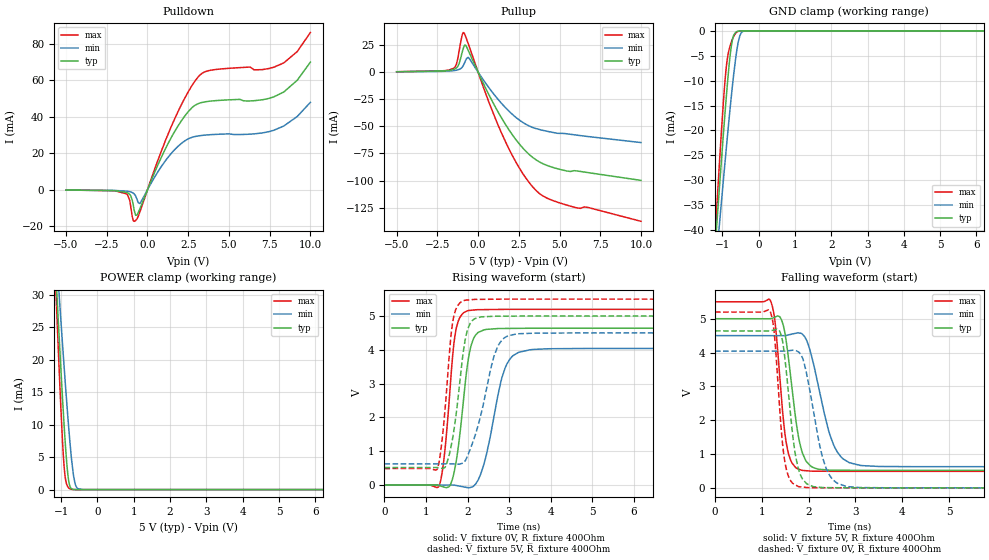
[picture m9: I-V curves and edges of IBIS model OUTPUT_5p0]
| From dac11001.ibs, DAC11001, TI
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|   OUTPUT_5p0 Model
[Model]   OUTPUT_5p0
Model_type   3-state
Polarity   Non-Inverting
Vmeas = 2.5
Vref = 0
Cref = 2pF
Rref = 100000
|   typ   min   max
C_comp   1.405pF   1.354pF   1.437pF
[Voltage Range]   5   4.5   5.5
[Temperature Range]   25   125   -40
[Pullup Reference]   5   4.5   5.5
[Pulldown Reference]   0   0   0
[Power Clamp Reference]   5   4.5   5.5
[GND Clamp Reference]   0   0   0
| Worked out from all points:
|   slope of the pulldown table from 0 to 0.75 V, typ, clamps not added: 47.3 ohm
|   slope of the pullup table from 0 to 0.75 V, typ, clamps not added: 32.1 ohm
|   GND clamp passes 1 mA (typ) near -0.69 V on its own axis
|   POWER clamp passes 1 mA (typ) near -0.78 V on its own axis
|   falling waveform, V_fixture 5V, R_fixture 400Ohm: 20-80 % time 253ps typ, 405ps min, 193ps max; typ from 5 V to 0.517 V
|   rising waveform, V_fixture 0V, R_fixture 400Ohm: 20-80 % time 262ps typ, 407ps min, 214ps max; typ from 0 V to 4.64 V
|   rising waveform, V_fixture 5V, R_fixture 400Ohm: 20-80 % time 272ps typ, 455ps min, 207ps max; typ from 0.517 V to 5 V
|   falling waveform, V_fixture 0V, R_fixture 400Ohm: 20-80 % time 222ps typ, 343ps min, 173ps max; typ from 4.64 V to 0 V
[Pulldown]
|   Voltage   I(typ)   I(min)   I(max)
-5V       -142.8uA   -116.5uA   -136.1uA
-1.25V    -1.527mA   -787.6uA   -2.341mA
-1.1V     -2.433mA   -1.025mA   -5.468mA
-875mV    -8.302mA   -1.831mA   -16.84mA
-725mV    -14.02mA   -3.432mA   -16.85mA
-455mV    -10.11mA   -7.363mA   -11.8mA
1.525V    29.73mA    20.64mA    36.03mA
2.41V     41.87mA    27.51mA    52.3mA
3.16V     47.45mA    29.62mA    62.48mA
7.75V     50.98mA    32.66mA    67.25mA
9.175V    59.95mA    40.1mA     75.72mA
10V       70.06mA    47.98mA    86.29mA
[GND Clamp]
|   Voltage   I(typ)   I(min)   I(max)
-5V       -455.7mA   -381.5mA   -546mA
-1.235V   -47.57mA   -51.99mA   -45.92mA
-1.13V    -36.77mA   -43.2mA    -32.86mA
-1.07V    -30.7mA    -38.23mA   -25.64mA
-950mV    -18.95mA   -28.46mA   -12.42mA
-875mV    -12.09mA   -22.52mA   -6.432mA
-785mV    -5.068mA   -15.68mA   -3.054mA
-725mV    -1.977mA   -11.41mA   -1.785mA
-590mV    -122.8uA   -3.502mA   -213.3uA
-485mV    -9.764uA   -489.6uA   -15.16uA
-275mV    0A         -1.303uA   0A
10V       0A         0A         0A
[Pullup]
|   Voltage   I(typ)   I(min)   I(max)
-5V       287.7uA    224.1uA    311.3uA
-1.49V    2.452mA    1.323mA    3.599mA
-1.325V   3.811mA    1.724mA    7.343mA
-1.16V    7.875mA    2.459mA    19.67mA
-965mV    18.82mA    4.665mA    34.63mA
-860mV    23.79mA    7.416mA    36.14mA
-575mV    19.02mA    13.11mA    24.9mA
1.48V     -43.28mA   -29.51mA   -57.5mA
2.365V    -63.08mA   -42.28mA   -84.07mA
3.37V     -78.83mA   -51.13mA   -106.1mA
5.05V     -89.77mA   -56.51mA   -120.7mA
10V       -99.8mA    -64.95mA   -137.5mA
[POWER Clamp]
|   Voltage   I(typ)   I(min)   I(max)
-5V       483.6mA    383.8mA    617mA
-1.145V   33.35mA    37.7mA     31.01mA
-1.13V    31.72mA    36.44mA    28.92mA
-1.1V     28.49mA    33.91mA    24.79mA
-1.055V   23.71mA    30.16mA    18.76mA
-965mV    14.52mA    22.8mA     7.888mA
-920mV    10.26mA    19.22mA    3.808mA
-830mV    3.216mA    12.37mA    580uA
-755mV    487.8uA    7.221mA    120.5uA
-620mV    6.266uA    1.055mA    4.234uA
-410mV    0A         3.37uA     0A
10V       0A         0A         0A
[Ramp]
R_load = 400
|   typ   min   max
dV/dt_r   2.78348/2.61903e-10   2.42479/4.06187e-10   3.11823/2.13547e-10
dV/dt_f   2.68951/2.52802e-10   2.32455/4.0158e-10   3.00713/1.92629e-10
[Falling Waveform]
V_fixture = 5V
V_fixture_min = 4.5V
V_fixture_max = 5.5V
R_fixture = 400Ohm
C_fixture = 0F
|   Time   V(typ)   V(min)   V(max)
0s        5V         4.5V       5.5V
1.179ns   5.001V     4.499V     5.548V
1.283ns   5.05V      4.499V     4.903V
1.423ns   4.957V     4.499V     2.609V
1.522ns   4.319V     4.507V     1.328V
1.738ns   1.895V     4.575V     585.1mV
1.859ns   1.07V      4.554V     519mV
2.634ns   522.1mV    1.02V      488.5mV
4.328ns   517.8mV    626.1mV    488.5mV
3.5us     517.5mV    625.7mV    488.1mV
[Rising Waveform]
V_fixture = 0V
V_fixture_min = 0V
V_fixture_max = 0V
R_fixture = 400Ohm
C_fixture = 0F
|   Time   V(typ)   V(min)   V(max)
0s        4.15nV     5.184pV    3.904nV
1.303ns   -10.72mV   1.617mV    -52.66mV
1.437ns   -60.16mV   1.783mV    817.1mV
1.58ns    -4.988mV   1.96mV     2.839V
1.778ns   1.125V     -24.2mV    4.852V
2.017ns   3.704V     -79.3mV    5.159V
2.169ns   4.389V     -4.845mV   5.18V
2.903ns   4.632V     3.452V     5.197V
4.935ns   4.639V     4.041V     5.197V
3.5us     4.639V     4.041V     5.197V
[Rising Waveform]
V_fixture = 5V
V_fixture_min = 4.5V
V_fixture_max = 5.5V
R_fixture = 400Ohm
C_fixture = 0F
|   Time   V(typ)   V(min)   V(max)
0s        517.5mV    625.7mV    488.1mV
1.269ns   518.7mV    627mV      462.5mV
1.395ns   492.5mV    627.2mV    1.401V
1.643ns   1.392V     627.4mV    4.811V
1.902ns   3.965V     657.4mV    5.451V
2.116ns   4.868V     1.229V     5.486V
2.612ns   4.991V     3.701V     5.497V
2.805ns   4.996V     4.248V     5.5V
4.608ns   5V         4.5V       5.5V
3.5us     5V         4.5V       5.5V
[Falling Waveform]
|Gnd
V_fixture = 0V
V_fixture_min = 0V
V_fixture_max = 0V
R_fixture = 400Ohm
C_fixture = 0F
|   Time   V(typ)   V(min)   V(max)
0s        4.639V     4.041V     5.197V
1.175ns   4.64V      4.04V      5.231V
1.266ns   4.67V      4.04V      4.564V
1.388ns   4.614V     4.04V      2.223V
1.494ns   3.806V     4.042V     752.7mV
1.672ns   1.412V     4.067V     123.3mV
1.793ns   508.3mV    4.01V      35.42mV
2.297ns   9.919mV    902.2mV    3.331mV
2.558ns   4.602mV    193.1mV    373.7uV
3.5us     -6.068nV   -385nV     -39.51nV
